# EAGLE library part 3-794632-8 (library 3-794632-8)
Rectangular Power Connectors, Header, Plug, Wire-to-Board, 8 Position, 3 mm [.118 in] Centerline, Printed Circuit Board, UL 94V-0, Micro MATE-N-LOK Source: Datasheet
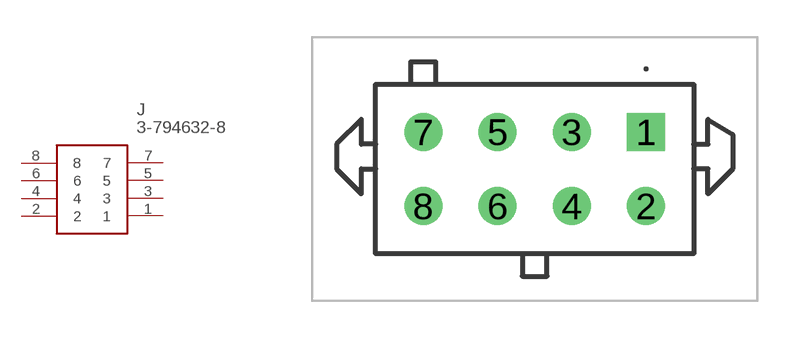
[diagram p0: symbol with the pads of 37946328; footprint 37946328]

Designator prefix J

## 3-794632-8 (Description: Rectangular Power Connectors, Header, Plug, Wire-to-Board, 8 Position, 3 mm [.118 in] Centerline, Printed Circuit Board, UL 94V-0, Micro MATE-N-LOK; Height: 9.44mm; Manufacturer_Name: TE Connectivity; Manufacturer_Part_Number: 3-794632-8; Mouser_Part_Number: 571-3-794632-8; Mouser_Price-Stock: https://www.mouser.co.uk/ProductDetail/TE-Connectivity-AMP/3-794632-8?qs=NgQsWEdBC4ddimdXLdgoFA%3D%3D)  [37946328]
1  1
2  2
3  3
4  4
5  5
6  6
7  7
8  8

## Footprint 37946328 (pad centres in mm)
3-794632-8-3
drill 1.02 pad 1.53 square: 1 0,0
drill 1.02 pad 1.53: 2 0,-3; 3 -3,0; 4 -3,-3; 5 -6,0; 6 -6,-3; 7 -9,0; 8 -9,-3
